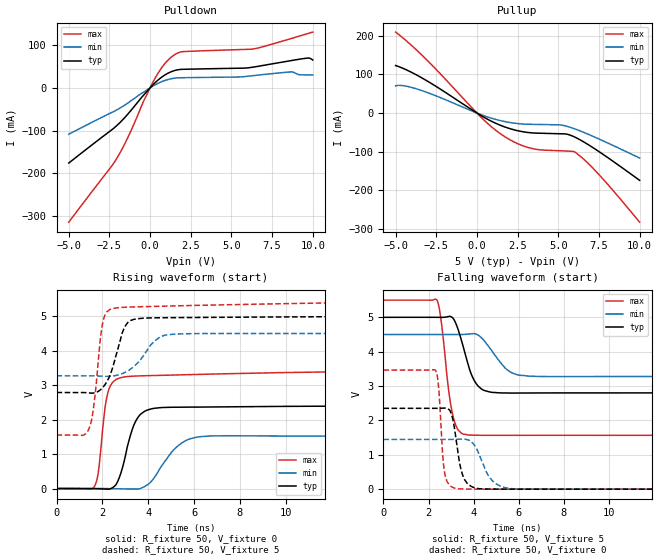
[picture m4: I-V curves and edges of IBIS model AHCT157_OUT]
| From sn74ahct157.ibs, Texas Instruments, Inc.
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[Model]   AHCT157_OUT
Model_type  Output
|Vref =   0.0
|Rref =   1000
Cref =   50p
Vmeas =   2.5
| variable   typ   min   max
C_comp   3.14pF   1.81pF   5.29pF
| C_pullup   3.06pF   1.93pF   4.48pF
| C_pulldown   3.22pF   1.81pF   5.29pF
[Temperature Range]   40   100   -40
| Ambient temperature   25   85   -40
[Voltage range]   5   4.5   5.5
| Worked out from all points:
|   slope of the pulldown table from 0 to 0.75 V, typ, clamps not added: 28.7 ohm
|   slope of the pullup table from 0 to 0.75 V, typ, clamps not added: 41 ohm
|   rising waveform, R_fixture 50, V_fixture 0: 20-80 % time 606ps typ, 995ps min, 376ps max; typ from 0 V to 2.4 V
|   falling waveform, R_fixture 50, V_fixture 5: 20-80 % time 615ps typ, 855ps min, 420ps max; typ from 5 V to 2.8 V
|   rising waveform, R_fixture 50, V_fixture 5: 20-80 % time 593ps typ, 914ps min, 375ps max; typ from 2.79 V to 5 V
|   falling waveform, R_fixture 50, V_fixture 0: 20-80 % time 361ps typ, 629ps min, 201ps max; typ from 2.35 V to 0 V
[Pulldown]
| AHCT157_OUT
|   Voltage   I(typ)   I(min)   I(max)
-5V       -176.3mA   -108.7mA   -315.1mA
-2.095V   -90.13mA   -52.7mA    -168.4mA
-1.395V   -62.76mA   -36.2mA    -118.7mA
-430mV    -18.36mA   -10.76mA   -33.93mA
245mV     9.806mA    5.708mA    18.29mA
800mV     27.48mA    15.8mA     51.72mA
1.35V     38.65mA    21.82mA    73.66mA
2.04V     43.57mA    23.89mA    85.15mA
6.4V      49.05mA    28.94mA    91.72mA
8.695V    64.14mA    37.44mA    115.9mA
9.74V     70mA       30.34mA    128mA
10V       65.43mA    30.34mA    130.9mA
[Pullup]
| AHCT157_OUT
|   Voltage   I(typ)   I(min)   I(max)
-5V       122.8mA    70.05mA    209.3mA
-4.43V    113.4mA    70.06mA    189.9mA
-3.445V   92.22mA    58.85mA    152.2mA
165mV     -4.355mA   -2.78mA    -7.196mA
1.145V    -26.36mA   -16.46mA   -44.25mA
2.165V    -42.12mA   -25.46mA   -72.31mA
3.185V    -50.56mA   -29.09mA   -89.58mA
5.11V     -53.66mA   -30.76mA   -97.66mA
5.54V     -54.78mA   -34.47mA   -98.42mA
6.03V     -62.54mA   -41.26mA   -101.2mA
7.465V    -98.77mA   -66.5mA    -157.5mA
10V       -174.1mA   -116.4mA   -282.3mA
[Ramp]
| AHCT157_OUT
| variable   typ   min   max
dV/dt_r   1.45/6.44E-10   0.93/1.09E-09   2.10/3.91E-10
dV/dt_f   1.34/6.41E-10   0.75/8.80E-10   2.38/4.26E-10
R_load = 50
[Rising Waveform]
| AHCT157_OUT
R_fixture =   50
C_fixture =   0
L_fixture =   0
V_fixture =   0
V_fixture_min = 0
V_fixture_max = 0
|   Time   V(typ)   V(min)   V(max)
0s        487.8uV    754.9uV    269.3uV
1.635ns   -1.388mV   916.4uV    40.51mV
1.815ns   -5.655mV   1.159mV    436.6mV
2.265ns   -16.81mV   -269.4uV   2.842V
2.66ns    195.9mV    -4.641mV   3.183V
3.045ns   1.074V     -10.63mV   3.248V
3.87ns    2.252V     68.22mV    3.275V
5.365ns   2.361V     1.276V     3.299V
6.69ns    2.368V     1.527V     3.321V
50ns      2.401V     1.51V      3.478V
[Falling Waveform]
| AHCT157_OUT
R_fixture =   50
C_fixture =   0
L_fixture =   0
V_fixture =   5
V_fixture_min = 4.5
V_fixture_max = 5.5
|   Time   V(typ)   V(min)   V(max)
0s        5V         4.5V       5.5V
2.38ns    5V         4.5V       5.493V
2.55ns    4.998V     4.5V       4.947V
2.885ns   5.022V     4.5V       2.915V
3.08ns    4.98V      4.5V       2.145V
3.755ns   3.631V     4.511V     1.577V
4.445ns   2.878V     4.338V     1.567V
5.515ns   2.797V     3.458V     1.567V
6.55ns    2.798V     3.286V     1.567V
50ns      2.797V     3.277V     1.564V
[Rising Waveform]
| AHCT157_OUT
R_fixture =   50
C_fixture =   0
L_fixture =   0
V_fixture =   5
V_fixture_min = 4.5
V_fixture_max = 5.5
|   Time   V(typ)   V(min)   V(max)
0s        2.788V     3.273V     1.553V
1.395ns   2.778V     3.272V     1.704V
1.615ns   2.774V     3.271V     2.348V
1.905ns   2.861V     3.264V     4.304V
2.04ns    2.952V     3.26V      4.88V
2.63ns    3.942V     3.288V     5.245V
3.195ns   4.867V     3.451V     5.268V
4.37ns    4.956V     4.327V     5.288V
5.175ns   4.961V     4.483V     5.301V
50ns      5V         4.5V       5.5V
[Falling Waveform]
| AHCT157_OUT
R_fixture =   50
C_fixture =   0
L_fixture =   0
V_fixture =   0
V_fixture_min = 0
V_fixture_max = 0
|   Time   V(typ)   V(min)   V(max)
0s        2.351V     1.446V     3.466V
2.31ns    2.352V     1.447V     3.459V
2.45ns    2.352V     1.446V     2.941V
2.725ns   2.359V     1.446V     440.5mV
3.045ns   2.114V     1.446V     61.52mV
3.325ns   985.1mV    1.452V     10.06mV
3.885ns   84.4mV     1.384V     1.35mV
4.785ns   3.349mV    280.4mV    -210.9uV
5.74ns    20.68uV    12.59mV    -32.46uV
50ns      485.3uV    738.4uV    276.3uV
